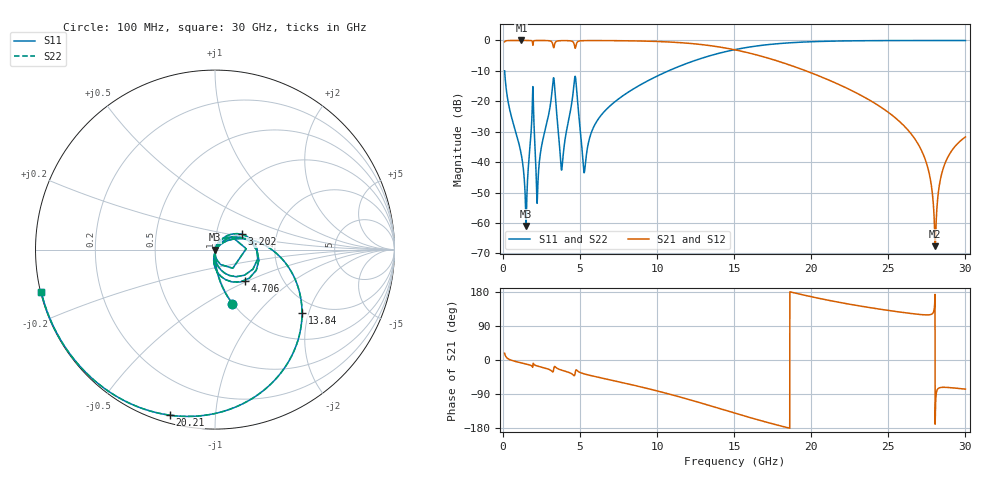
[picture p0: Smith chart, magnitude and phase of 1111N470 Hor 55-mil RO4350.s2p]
# GHz S MA R 50
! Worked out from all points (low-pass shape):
!   3201 points, 100 MHz to 30 GHz, reference 50 ohm
!   highest |S21| = -0.01 dB at 1.193 GHz (marker M1); lowest = -67.6 dB at 28.05 GHz (marker M2)
!   |S21| within 3 dB of the highest: start of sweep to 14.97 GHz
!   lowest |S11| = -61.0 dB at 1.492 GHz (marker M3), VSWR 1.00, Z = 50.1 - j0.0184 ohm
!   |S11| at or under -10 dB: 100.2 MHz to 10.73 GHz (10.63 GHz wide, 196 % of centre)
!   |S22| runs from -61.0 to 0.0 dB; largest |S21 - S12| = 0
!   S11 on the Smith chart (normalised r, x): 100 MHz: 0.99, -0.67; 3.202 GHz: 1.32, +0.23; 4.706 GHz: 1.30, -0.48; 13.84 GHz: 1.64, -1.81; 20.21 GHz: 0.04, -0.76; 30 GHz: 0.00, -0.12
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0.1  0.3169 -72.2  0.9482 17.8  0.9482 17.8  0.3169 -72.2
1.193219  0.01285 -94.8  0.9991 -7.8  0.9991 -7.8  0.01285 -94.8
1.492219  0.0008898 -11.9  0.9989 -10.6  0.9989 -10.6  0.0008898 -11.9
1.875312  0.05827 59.1  0.9838 -16.6  0.9838 -16.6  0.05827 59.1
2.26775  0.004904 51.5  0.9979 -16.3  0.9979 -16.3  0.004904 51.5
3.202125  0.171 30.0  0.9059 -31.2  0.9059 -31.2  0.171 30.0
3.360969  0.1527 -64.6  0.8898 -17.2  0.8898 -17.2  0.1527 -64.6
3.818812  0.007797 -1.1  0.9925 -27.0  0.9925 -27.0  0.007797 -1.1
4.706469  0.2398 -46.3  0.7682 -28.7  0.7682 -28.7  0.2398 -46.3
5.089563  0.02054 -94.0  0.9889 -34.4  0.9889 -34.4  0.02054 -94.0
5.304469  0.007633 0.2  0.9933 -37.1  0.9933 -37.1  0.007633 0.2
6.435062  0.06206 39.5  0.9945 -47.9  0.9945 -47.9  0.06206 39.5
10.06978  0.2648 7.0  0.96 -82.4  0.96 -82.4  0.2648 7.0
13.84466  0.5997 -36.0  0.7939 -125.6  0.7939 -125.6  0.5997 -36.0
15.05  0.7066 -50.7  0.7004 -140.3  0.7004 -140.3  0.7066 -50.7
20.03956  0.9529 -103.8  0.29 166.6  0.29 166.6  0.9529 -103.8
20.20775  0.9562 -105.2  0.279 165.1  0.279 165.1  0.9562 -105.2
25.01978  0.9946 -140.0  0.06519 130.7  0.06519 130.7  0.9946 -140.0
27.22491  0.9967 -152.5  0.01416 119.5  0.01416 119.5  0.9967 -152.5
28.04716  0.9968 -156.8  0.0004151 -148.8  0.0004151 -148.8  0.9968 -156.8
28.6545  0.9968 -159.8  0.009199 -72.1  0.009199 -72.1  0.9968 -159.8
30  0.9965 -166.3  0.02592 -76.9  0.02592 -76.9  0.9965 -166.3
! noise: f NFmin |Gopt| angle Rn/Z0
0.1  0.000684  0.7411  1.581  0.0005296
3.417  0.05634  0.8851  24.1  0.1018
6.743  0.01895  0.4859  45.11  0.00549
10.06  0.02522  0.4597  61.87  0.006055
13.39  0.03667  0.5214  77.13  0.008721
16.7  0.05737  0.6345  93.52  0.01465
20.03  0.1023  0.7709  112.1  0.02942
23.35  0.2304  0.8911  131.5  0.07915
26.67  1.079  0.9754  149.8  0.6877
30  1.057  0.9742  166.2  0.1371
